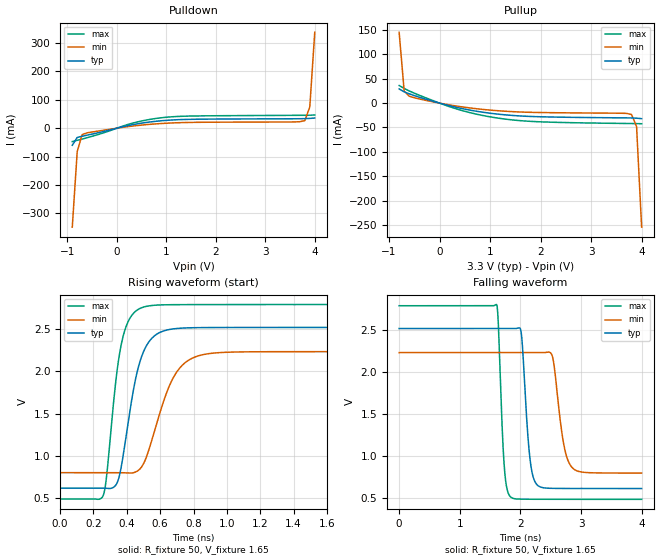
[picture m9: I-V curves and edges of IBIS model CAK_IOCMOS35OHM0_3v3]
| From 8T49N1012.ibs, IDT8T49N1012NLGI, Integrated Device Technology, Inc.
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| 4.00000e+00   -8.62883e-03   -4.17625e-01   -1.64224e-03
| 4.10000e+00   -1.92677e-02   -6.96871e-01   -7.13120e-03
| 4.20000e+00   -1.63537e-01   -9.76499e-01   -1.62698e-02
| 4.30000e+00   -5.37186e-01   -1.25639e+00   -2.58184e-02
| 4.40000e+00   -9.11197e-01   -1.53649e+00   -5.42192e-02
| 4.50000e+00   -1.28553e+00   -1.81678e+00   -4.53522e-01
| 4.60000e+00   -1.66015e+00   -2.09725e+00   -9.32352e-01
| 4.70000e+00   -2.03503e+00   -2.37789e+00   -1.41151e+00
| 4.80000e+00   -2.41015e+00   -2.65869e+00   -1.89093e+00
| 4.90000e+00   -2.78547e+00   -2.93964e+00   -2.37058e+00
| 5.00000e+00   -3.16097e+00   -3.22073e+00   -2.85041e+00
| 5.10000e+00   -3.53662e+00   -3.50195e+00   -3.33037e+00
| 5.20000e+00   -3.91240e+00   -3.78329e+00   -3.81046e+00
| 5.30000e+00   -4.28830e+00   -4.06475e+00   -4.29065e+00
| 5.40000e+00   -4.66429e+00   -4.34631e+00   -4.77094e+00
| 5.50000e+00   -5.04036e+00   -4.62797e+00   -5.25130e+00
| 5.60000e+00   -5.41651e+00   -4.90972e+00   -5.73173e+00
| 5.70000e+00   -5.79271e+00   -5.19155e+00   -6.21221e+00
| 5.80000e+00   -6.16897e+00   -5.47346e+00   -6.69272e+00
| 5.90000e+00   -6.54526e+00   -5.75544e+00   -7.17325e+00
| 6.00000e+00   -6.92159e+00   -6.03748e+00   -7.65380e+00
| 6.10000e+00   -7.29795e+00   -6.31959e+00   -8.13435e+00
| 6.20000e+00   -7.67433e+00   -6.60175e+00   -8.61491e+00
| 6.30000e+00   -8.05073e+00   -6.88396e+00   -9.09546e+00
| 6.40000e+00   -8.42715e+00   -7.16622e+00   -9.57600e+00
| 6.50000e+00   -8.80357e+00   -7.44852e+00   -1.00565e+01
| 6.60000e+00   -9.18001e+00   -7.73087e+00   -1.05371e+01
[Model] CAK_IOCMOS35OHM0_3v3
Model_type   Output
Polarity   Non-Inverting
|   typ   min   max
C_comp   2pF   1.5pF   2.5pF
Vmeas = 1.65V
Rref = 50
Cref = 0
Vref = 1.65V
|   typ   min   max
[Voltage range]   3.3V   3.135V   3.465V
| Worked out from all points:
|   slope of the pulldown table from 0 to 0.495 V, typ, clamps not added: 28 ohm
|   slope of the pullup table from 0 to 0.495 V, typ, clamps not added: 40.4 ohm
|   rising waveform, R_fixture 50, V_fixture 1.65: 20-80 % time 105ps typ, 150ps min, 79.5ps max; typ from 0.616 V to 2.52 V
|   falling waveform, R_fixture 50, V_fixture 1.65: 20-80 % time 105ps typ, 152ps min, 78.2ps max; typ from 2.52 V to 0.616 V
[Pulldown]
|Voltage   I (typ)   I (min)   I (max)
|Note, modeling breaks down at 250mA and above.  This is well beyond the functional   |
|operating range of the device.  Should this scenario occur, catastrophic failure and   |
|possible damage to the device and/or board is of higher concern than the I-V curve   |
|behavior.  The IBIS checker will flag currents in excess of 10A with warnings.  Lines   |
|with currents in excess of 0.35 A have been commented out.  The points still remain|
|available to the user if the user desires to use them.   |
|-3.200000e+00   -8.493290e+00   -6.714440e+00   -1.050260e+01
|-3.100000e+00   -8.124360e+00   -6.438000e+00   -1.003100e+01
|-3.000000e+00   -7.755410e+00   -6.161480e+00   -9.559400e+00
|-2.900000e+00   -7.386440e+00   -5.884870e+00   -9.087740e+00
|-2.800000e+00   -7.017440e+00   -5.608380e+00   -8.616030e+00
|-2.700000e+00   -6.648410e+00   -5.331790e+00   -8.144420e+00
|-2.600000e+00   -6.279330e+00   -5.055300e+00   -7.672720e+00
|-2.500000e+00   -5.910310e+00   -4.778710e+00   -7.201020e+00
|-2.400000e+00   -5.541320e+00   -4.502120e+00   -6.729300e+00
|-2.300000e+00   -5.172160e+00   -4.225510e+00   -6.257560e+00
|-2.200000e+00   -4.803070e+00   -3.948880e+00   -5.785780e+00
|-2.100000e+00   -4.433930e+00   -3.672220e+00   -5.313960e+00
|-2.000000e+00   -4.064730e+00   -3.395520e+00   -4.842060e+00
|-1.900000e+00   -3.695480e+00   -3.118780e+00   -4.370190e+00
|-1.800000e+00   -3.326160e+00   -2.842010e+00   -3.898200e+00
|-1.700000e+00   -2.956770e+00   -2.565190e+00   -3.426120e+00
|-1.600000e+00   -2.587290e+00   -2.288330e+00   -2.953930e+00
|-1.500000e+00   -2.217720e+00   -2.011420e+00   -2.481610e+00
|-1.400000e+00   -1.848050e+00   -1.734440e+00   -2.009140e+00
|-1.300000e+00   -1.478260e+00   -1.457420e+00   -1.536510e+00
|-1.200000e+00   -1.108350e+00   -1.180340e+00   -1.063690e+00
|-1.100000e+00   -7.383240e-01   -9.031900e-01   -5.906750e-01
|-1.000000e+00   -3.681570e-01   -6.259730e-01   -1.221630e-01
-900mV    -60.19mA   -348.7mA   -47.03mA
-800mV    -32.42mA   -81.9mA    -42.64mA
-700mV    -28.27mA   -22.55mA   -38.23mA
-600mV    -24.51mA   -16.26mA   -33.47mA
300mV     11.82mA    7.229mA    17.01mA
900mV     26.25mA    16.56mA    36.87mA
1.5V      31.35mA    20.45mA    42.88mA
3.6V      33.33mA    22.16mA    45.4mA
3.8V      33.77mA    26.83mA    45.62mA
3.9V      34.57mA    75.14mA    45.83mA
4V        35.86mA    337.9mA    46.52mA
|4.100000e+00   3.848030e-02   6.224830e-01   4.781350e-02
|4.200000e+00   9.082200e-02   9.071100e-01   4.966550e-02
|4.300000e+00   4.538650e-01   1.191800e+00   5.150950e-02
|4.400000e+00   8.340300e-01   1.476560e+00   5.960320e-02
|4.500000e+00   1.214320e+00   1.761400e+00   3.674390e-01
|4.600000e+00   1.594730e+00   2.046320e+00   8.538500e-01
|4.700000e+00   1.975260e+00   2.331310e+00   1.340450e+00
|4.800000e+00   2.355930e+00   2.616390e+00   1.827250e+00
|4.900000e+00   2.736740e+00   2.901550e+00   2.314260e+00
|5.000000e+00   3.117710e+00   3.186820e+00   2.801510e+00
|5.100000e+00   3.498840e+00   3.472180e+00   3.288990e+00
|5.200000e+00   3.880160e+00   3.757660e+00   3.776730e+00
|5.300000e+00   4.261650e+00   4.043240e+00   4.264740e+00
|5.400000e+00   4.643360e+00   4.328950e+00   4.753000e+00
|5.500000e+00   5.025310e+00   4.614810e+00   5.241510e+00
|5.600000e+00   5.407480e+00   4.900780e+00   5.730390e+00
|5.700000e+00   5.789830e+00   5.186980e+00   6.219440e+00
|5.800000e+00   6.172460e+00   5.473260e+00   6.708650e+00
|5.900000e+00   6.555470e+00   5.759810e+00   7.198040e+00
|6.000000e+00   6.938650e+00   6.046500e+00   7.687410e+00
|6.100000e+00   7.322090e+00   6.333420e+00   8.176760e+00
|6.200000e+00   7.705790e+00   6.620650e+00   8.665980e+00
|6.300000e+00   8.089710e+00   6.907970e+00   9.155080e+00
|6.400000e+00   8.473860e+00   7.195650e+00   9.643830e+00
|6.500000e+00   8.857910e+00   7.483570e+00   1.013240e+01
|6.600000e+00   9.242030e+00   7.771810e+00   1.062080e+01
[Pullup]
|Voltage   I (typ)   I (min)   I (max)
|Note, modeling breaks down at 250mA and above.  This is well beyond the functional   |
|operating range of the device.  Should this scenario occur, catastrophic failure and   |
|possible damage to the device and/or board is of higher concern than the I-V curve   |
|behavior.  The IBIS checker will flag currents in excess of 10A with warnings.  Lines   |
|with currents in excess of 0.35 A have been commented out.  The points still remain|
|available to the user if the user desires to use them.   |
|-3.200000e+00   8.853810e+00   7.014990e+00   1.093020e+01
|-3.100000e+00   8.472360e+00   6.729060e+00   1.044250e+01
|-3.000000e+00   8.090810e+00   6.443210e+00   9.954900e+00
|-2.900000e+00   7.709190e+00   6.157270e+00   9.467260e+00
|-2.800000e+00   7.327490e+00   5.871240e+00   8.979350e+00
|-2.700000e+00   6.945650e+00   5.585260e+00   8.491310e+00
|-2.600000e+00   6.563570e+00   5.299130e+00   8.002840e+00
|-2.500000e+00   6.181360e+00   5.012980e+00   7.514440e+00
|-2.400000e+00   5.799130e+00   4.726490e+00   7.026020e+00
|-2.300000e+00   5.416880e+00   4.440050e+00   6.537590e+00
|-2.200000e+00   5.034710e+00   4.153630e+00   6.049220e+00
|-2.100000e+00   4.652590e+00   3.867250e+00   5.560820e+00
|-2.000000e+00   4.270460e+00   3.580890e+00   5.072480e+00
|-1.900000e+00   3.888340e+00   3.294560e+00   4.584130e+00
|-1.800000e+00   3.506230e+00   3.008250e+00   4.095780e+00
|-1.700000e+00   3.124140e+00   2.721960e+00   3.607430e+00
|-1.600000e+00   2.742050e+00   2.435680e+00   3.119060e+00
|-1.500000e+00   2.359970e+00   2.149430e+00   2.630680e+00
|-1.400000e+00   1.977880e+00   1.863180e+00   2.142280e+00
|-1.300000e+00   1.595790e+00   1.576950e+00   1.653860e+00
|-1.200000e+00   1.213680e+00   1.290720e+00   1.165390e+00
|-1.100000e+00   8.315400e-01   1.004480e+00   6.768650e-01
|-1.000000e+00   4.493550e-01   7.182370e-01   1.882560e-01
|-9.000000e-01   8.408600e-02   4.319150e-01   4.210040e-02
-800mV    29.05mA    145.3mA    36.1mA
-700mV    23.14mA    24.2mA     30.12mA
-600mV    19.05mA    14.08mA    24.97mA
-200mV    5.933mA    4.128mA    7.978mA
300mV     -7.936mA   -5.456mA   -10.8mA
700mV     -16.15mA   -11.14mA   -21.94mA
1.2V      -23.1mA    -15.97mA   -31.42mA
2V        -28.01mA   -19.3mA    -38.4mA
3.6V      -30.21mA   -20.74mA   -41.65mA
3.8V      -30.44mA   -23.34mA   -41.88mA
3.9V      -30.91mA   -48.13mA   -42.01mA
4V        -31.87mA   -254.5mA   -42.33mA
|4.100000e+00   -3.367380e-02   -5.304420e-01   -4.331370e-02
|4.200000e+00   -5.946600e-02   -8.064000e-01   -4.489090e-02
|4.300000e+00   -3.657020e-01   -1.082400e+00   -4.653200e-02
|4.400000e+00   -7.343440e-01   -1.358440e+00   -5.131470e-02
|4.500000e+00   -1.103040e+00   -1.634500e+00   -2.815040e-01
|4.600000e+00   -1.471790e+00   -1.910610e+00   -7.530450e-01
|4.700000e+00   -1.840590e+00   -2.186740e+00   -1.224640e+00
|4.800000e+00   -2.209440e+00   -2.462910e+00   -1.696310e+00
|4.900000e+00   -2.578330e+00   -2.739100e+00   -2.168030e+00
|5.000000e+00   -2.947260e+00   -3.015330e+00   -2.639810e+00
|5.100000e+00   -3.316250e+00   -3.291590e+00   -3.111640e+00
|5.200000e+00   -3.685290e+00   -3.567890e+00   -3.583550e+00
|5.300000e+00   -4.054380e+00   -3.844230e+00   -4.055520e+00
|5.400000e+00   -4.423530e+00   -4.120620e+00   -4.527570e+00
|5.500000e+00   -4.792740e+00   -4.397050e+00   -4.999680e+00
|5.600000e+00   -5.162060e+00   -4.673530e+00   -5.471950e+00
|5.700000e+00   -5.531420e+00   -4.950020e+00   -5.944350e+00
|5.800000e+00   -5.900910e+00   -5.226650e+00   -6.416820e+00
|5.900000e+00   -6.270430e+00   -5.503370e+00   -6.889450e+00
|6.000000e+00   -6.640110e+00   -5.780090e+00   -7.362260e+00
|6.100000e+00   -7.009940e+00   -6.056930e+00   -7.835260e+00
|6.200000e+00   -7.379840e+00   -6.333780e+00   -8.308360e+00
|6.300000e+00   -7.750010e+00   -6.610850e+00   -8.781870e+00
|6.400000e+00   -8.120260e+00   -6.887950e+00   -9.255490e+00
|6.500000e+00   -8.490690e+00   -7.165180e+00   -9.729400e+00
|6.600000e+00   -8.861410e+00   -7.442550e+00   -1.020370e+01
[Ramp]
|   typ   min   max
dV/dt_r   1.147/0.105n   0.865/0.15n   1.387/0.079n
dV/dt_f   1.149/0.105n   0.865/0.152n   1.393/0.078n
R_load =   50.0000
[Rising Waveform]
R_fixture = 50
V_fixture = 1.65   |Vcc_typ
V_fixture_min = 1.5675 |Vcc_min
V_fixture_max = 1.7325 |Vcc_max
C_fixture = 0.0p
| Time   typ   min   max
0s        615.5mV    799.2mV    486.9mV
257.8ps   615.7mV    799.2mV    524.6mV
280ps     612.9mV    799.3mV    780.9mV
333.3ps   650mV      799.5mV    1.877V
368.9ps   894.4mV    798.6mV    2.342V
444.4ps   1.832V     801.2mV    2.7V
502.2ps   2.244V     913.2mV    2.766V
680ps     2.506V     1.931V     2.793V
866.7ps   2.521V     2.204V     2.794V
4ns       2.523V     2.236V     2.795V
[Falling Waveform]
R_fixture = 50
V_fixture = 1.65   |Vcc_typ
V_fixture_min = 1.5675 |Vcc_min
V_fixture_max = 1.7325 |Vcc_max
C_fixture = 0.0p
| Time   typ   min   max
0s        2.523V     2.236V     2.795V
1.609ns   2.523V     2.236V     2.807V
1.733ns   2.523V     2.236V     887.2mV
1.844ns   2.523V     2.236V     511.7mV
2.009ns   2.495V     2.236V     488.9mV
2.147ns   1.048V     2.236V     487.9mV
2.267ns   666.9mV    2.236V     487.6mV
2.524ns   617.9mV    2.199V     487.3mV
2.849ns   616.2mV    869.5mV    487.1mV
4ns       615.6mV    799.6mV    486.9mV
